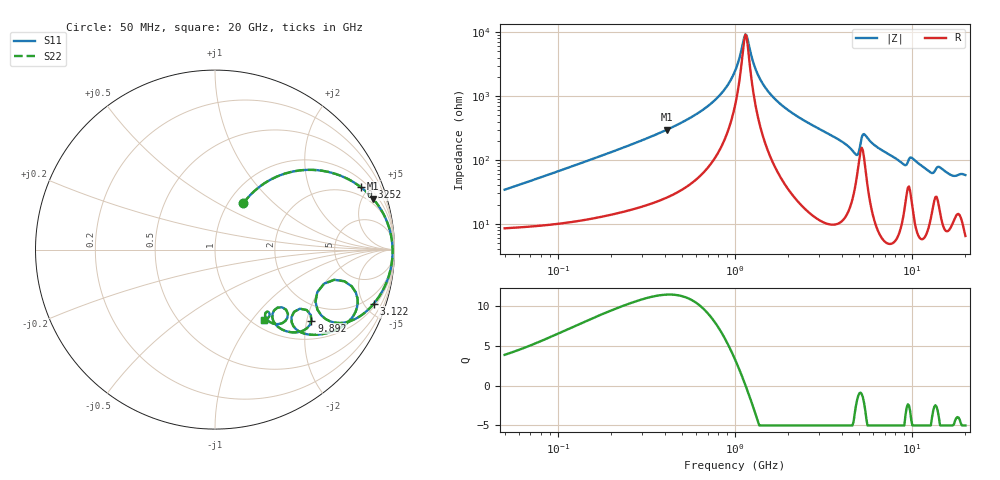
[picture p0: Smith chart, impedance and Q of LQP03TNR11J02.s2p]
!Murata Part Number: LQP03TNR11J02
!These Parameters are Measured in Series Mode Connection
!  o--[Z]--o
!Port1  Port2
!  o-------o
!Freq. Start=50[MHz] Stop=20[GHz], 401[Steps]
# Hz S RI R 50
!Freq.(Hz) S11(Real) S11(Imag) S21(Real) S21(Imag) S12(Real) S12(Imag) S22(Real) S22(Imag)
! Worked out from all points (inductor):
!   401 points, 50 MHz to 20 GHz, reference 50 ohm
!   read as one part in series: L = 105 nH near 51.52 MHz
!   highest Q = 11.5 at 413.2 MHz (marker M1), where L = 115 nH
!   self-resonance near 1.144 GHz
!   S11 on the Smith chart (normalised r, x): 50 MHz: 1.17, +0.67; 325.2 MHz: 1.40, +4.47; 3.122 GHz: 1.22, -5.76; 9.892 GHz: 1.49, -2.13; 20 GHz: 1.13, -1.16
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5e7  0.1579 0.2582  0.8421 -0.2582  0.8421 -0.2582  0.1579 0.2582
1.364002e8  0.4555 0.4388  0.5445 -0.4388  0.5445 -0.4388  0.4555 0.4388
3.251725e8  0.8134 0.3472  0.1866 -0.3472  0.1866 -0.3472  0.8134 0.3472
3.721004e8  0.853 0.3129  0.147 -0.3129  0.147 -0.3129  0.853 0.3129
4.132341e8  0.8797 0.2847  0.1203 -0.2847  0.1203 -0.2847  0.8797 0.2847
7.411344e8  0.9704 0.1205  0.0296 -0.1205  0.0296 -0.1205  0.9704 0.1205
1e9  0.987 0.0379  0.013 -0.0379  0.013 -0.0379  0.987 0.0379
1.127304e9  0.9892 0.00509  0.0108 -0.00509  0.0108 -0.00509  0.9892 0.00509
1.161586e9  0.9894 -0.00314  0.0106 0.00314  0.0106 0.00314  0.9894 -0.00314
1.309461e9  0.9886 -0.0362  0.0114 0.0362  0.0114 0.0362  0.9886 -0.0362
1.521052e9  0.9842 -0.0783  0.0158 0.0783  0.0158 0.0783  0.9842 -0.0783
2.728004e9  0.917 -0.2571  0.083 0.2571  0.083 0.2571  0.917 -0.2571
3.121702e9  0.8836 -0.3025  0.1164 0.3025  0.1164 0.3025  0.8836 -0.3025
4.677679e9  0.6165 -0.3871  0.3835 0.3871  0.3835 0.3871  0.6165 -0.3871
5.194772e9  0.7208 -0.1763  0.2792 0.1763  0.2792 0.1763  0.7208 -0.1763
5.598765e9  0.7905 -0.3251  0.2095 0.3251  0.2095 0.3251  0.7905 -0.3251
7.442007e9  0.5935 -0.4716  0.4065 0.4716  0.4065 0.4716  0.5935 -0.4716
9.041845e9  0.4272 -0.405  0.5728 0.405  0.5728 0.405  0.4272 -0.405
9.892087e9  0.5369 -0.396  0.4631 0.396  0.4631 0.396  0.5369 -0.396
1.257102e10  0.3242 -0.3961  0.6758 0.3961  0.6758 0.3961  0.3242 -0.3961
1.417136e10  0.403 -0.3811  0.597 0.3811  0.597 0.3811  0.403 -0.3811
2e10  0.2748 -0.3939  0.7252 0.3939  0.7252 0.3939  0.2748 -0.3939
